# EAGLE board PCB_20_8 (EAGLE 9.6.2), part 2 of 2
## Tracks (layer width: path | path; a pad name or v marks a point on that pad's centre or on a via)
1PPS
  Top 0.406: U$1.4_TIMEPULSE 26.67,99.18 27.94,100.33 R703.2
+3V3  (via drill 0.3, 0.61)
  Top 0.152: IC800.57 IC800.58
  Top 0.254: v105.41,29.84 105.41,27.94 R825.2 | v105.41,37.47 107.95,37.47 | 114.16,61.42 IC800.19 | IC800.11 115.25,57.42 115.25,57.25 C805.1 | 97.37,52.42 IC800.75 | R821.1 85.41,57.47 v85.41,50.48 R822.1 | 111.76,87 111.76,87.02 | 114.94,60.64 C800.1 | v118.07,48.9 R803.2 120.44,41.35 BOOT0.1 | 99.41,60.96 99.41,60.92 IC800.58
  Top 0.305: 114.16,61.42 114.94,60.64 | v111.68,68.9 110.41,68.9 IC800.28 110.41,61.42 | 111.41,45.94 111.41,42.23 107.95,42.23 107.95,37.47 SERIAL.2 | 97.37,52.42 v97.37,50.48 C801.1 C817.1 97.37,40.01 SWD.1 | IC800.11 110.09,57.42 | 99.38,53.66 99.38,52.42 IC800.75 | 99.38,53.66 99.38,60.96 99.41,60.96 | 99.41,60.96 | 99.41,60.96 IC800.50 99.41,68.9 v98.42,68.9 C803.1 | IC800.19 110.41,61.42 | 110.09,53.66 110.49,53.34 111.41,52.42 IC800.100 v111.41,48.9 111.41,47.31 | 110.09,57.42 110.09,53.66 | 110.09,57.42 110.09,61.42 110.41,61.42 | 111.41,47.31 111.41,45.94 | 111.41,45.94 C802.1 | C804.1 111.76,68.9 | C815.1 111.76,71.12 | C816.1 111.51,47.41 111.41,47.31 | 110.09,53.66 99.38,53.66
  Top 0.406: 111.76,82.91 111.76,77.79 | 111.76,77.79 111.76,71.12 111.76,68.9 v111.68,68.9 | 111.76,82.91 111.76,87.02 IC502.3 | C510.1 111.76,87 | BOOT1.3 111.76,82.91 | F800.2 111.76,77.79
  Bottom 0.254: v105.41,29.84 v105.41,37.47 | v85.41,50.48 v97.37,50.48 | v118.07,48.9 v111.41,48.9
  Bottom 0.305: v111.68,68.9 v98.42,68.9 | BOOT0.2 BOOT0.1
  Bottom 0.406: BOOT1.4 BOOT1.3
+3V3-C  (via drill 0.61)
  Top 0.406: D3-C.2 v156.21,118.43 D4-C.2 | D6-C.2 v162.56,118.43 D5-C.2 | D1-C.2 v149.86,118.43 D2-C.2 | IC4.3 v162.88,104.14 162.24,105.41 IC3.7 | IC3.3 v153.03,104.14 152.4,105.41 IC2.7 | IC2.3 v142.56,104.14 142.56,92.98 C15.1 C9.1 147.64,90.79 IC5.5 | v172.72,104.14 172.72,105.41 IC4.7
  Bottom 0.406: v162.56,118.43 v156.21,118.43 153.67,118.43 | v172.72,104.14 v162.88,104.14 153.67,104.14 | 153.67,104.14 v153.03,104.14 v142.56,104.14 | v149.86,118.43 153.67,118.43 | 153.67,118.43 153.67,104.14
+3V3-E  (via drill 0.3, 0.5)
  Top 0.254: IC600.20 IC600.19
  Top 0.305: R607.2 101.6,100.75 v101.6,102.87
  Top 0.406: 86.36,115.25 v86.36,112.08 86.36,110.49 | 86.36,110.49 91.44,110.49 | v73.03,110.49 86.36,110.49 | v99.06,110.49 IC600.19 | IC600.25 91.44,110.49 | 91.44,110.49 v99.06,110.49 | v106.68,112.08 106.68,121.92 106.68,124.46 C606.2 IC504.3 | IC600.28 86.36,115.25 | 86.36,115.25 C604.2 | IC600.15 104.14,110.49 v101.6,110.49 v99.06,110.49 | F600.1 v43.18,110.49
  Bottom 0.305: v101.6,102.87 v101.6,110.49
  Bottom 0.406: v43.18,110.49 v73.03,110.49 | v106.68,112.08 v86.36,112.08
+3V3-G
  Top 0.406: F700.1 C518.1 45.24,104.87 IC505.3
+5V  (via drill 0.3 pad 0.25, 0.35, 0.6)
  Top 0.254: v59.05,12.38 C419.2 53.34,13.26 53.02,14.29 IC403.7 | IC303.7 53.02,35.24 | 53.02,56.52 IC203.7 | IC103.7 53.02,78.11
  Top 0.305: 53.02,35.24 53.34,34.21 C319.2 v59.05,33.34 59.05,30.58 C227.2 IC304.5 | 53.02,56.52 53.34,55.48 C219.2 v59.05,54.61 59.05,51.85 C327.2 IC204.5 | 53.02,78.11 53.34,77.08 C119.2 v59.05,76.2 59.05,73.44 C427.2 IC104.5 | v59.05,12.38 59.05,9.63 C127.2 IC404.5
  Top 0.406: v75.25,80.01 v75.25,70.8 v75.25,58.42 v75.25,37.15 v75.25,16.19 v75.25,12.7 v75.25,6.99 | v90.17,7.94 C513.1 97.16,7.95 IC503.5 | L403.1 v11.43,12.7 | v90.17,12.7 87.32,12.69 v86.36,12.7
  Bottom 0.305: v75.25,16.19 62.87,16.19 62.87,12.38 v59.05,12.38 | v59.05,33.34 62.87,33.34 62.87,37.15 v75.25,37.15 | v59.05,54.61 62.87,54.61 62.87,58.42 v75.25,58.42 | v59.05,76.2 62.87,76.2 62.87,80.01 v75.25,80.01
  Bottom 0.406: v75.25,70.8 16.51,70.8 H-INPUT.4 | H-INPUT.4 | v75.25,6.99 74.61,6.35 11.43,6.35 v11.43,12.7 | v86.36,12.7 | v75.25,12.7 | v86.36,12.7 v75.25,12.7 | v90.17,12.7 v90.17,7.94
A1
  Top 0.406: R17.1 R10.1 IC4.4
A2
  Top 0.406: R15.1 R8.1 IC3.4
A3
  Top 0.305: 146.05,102.73 IC2.4
  Top 0.406: R12.1 R7.1 146.05,102.73
ADA4891
  Top 0.406: IC1.1 160.66,26.04 160.66,27.94 IC1.4 R2.1 R5.1
AGND  (via drill 0.3, 0.5, 0.6, 0.6 pad 0.25)
  Top 0.254: IC103.3 IC103.2 53.02,86.04 54.61,87.23 C118.2 | 24.45,81.92 29.84,81.92 C105.1 30.8,79.38 32.07,79.38 | IC203.3 IC203.2 53.02,64.45 54.61,65.64 C218.2 | IC202.4 47.82,59.05 45.72,59.05 C214.2 44.45,57.7 v44.45,55.24 | 24.45,38.73 24.45,39.05 29.84,39.05 C305.1 30.8,36.51 32.07,36.51 | 24.45,38.73 C304.1 24.13,36.73 C300.2 C301.2 18.73,33.72 v18.73,33.34 17.78,32.38 R305.1 | R302.2 24.45,38.73 | C401.2 | C401.2 C400.2 24.13,15.77 C404.1 24.45,18.1 | C106.1 C107.1 39.05,71.75 43.5,71.75 R115.1 45.51,72.81 v45.72,73.03 | C406.1 C407.1 39.05,7.94 43.81,7.94 R415.1 46.26,9.27 v46.35,9.21 | C306.1 C307.1 39.05,28.89 43.5,28.89 R315.1 45.67,30.19 v45.72,30.16 | IC403.3 IC403.2 53.02,22.23 54.61,23.42 C418.2 | IC303.3 IC303.2 53.02,43.18 54.61,44.37 C318.2 | 56.83,84.77 v55.88,86.04 55.88,88.03 C118.2 | 56.83,41.91 v55.88,43.18 55.88,45.17 C318.2 | 56.83,20.95 v55.88,22.23 55.88,24.21 C418.2 | v63.5,84.77 56.83,84.77 | v63.5,63.18 56.83,63.18 | 56.83,63.18 v55.88,64.45 55.88,66.36 54.61,66.36 C218.2 | v63.5,41.91 56.83,41.91 | v63.5,20.95 56.83,20.95 | R105.1 17.78,75.25 v18.73,76.2 18.73,76.58 C101.2 C100.2 24.13,79.59 C104.1 24.45,81.92 | R205.1 17.78,53.66 v18.73,54.61 18.73,54.99 C201.2 C200.2 24.13,58 C204.1 24.45,60.01 | R309.1 32.07,36.51 | 32.07,36.51 36.51,36.51 | R310.1 38.73,36.51 36.51,36.51 | 36.51,36.51 R308.1 38.42,33.76 R311.1 38.73,33.97 40.96,33.97 | 24.45,60.01 24.45,60.33 29.84,60.33 C205.1 30.8,57.78 32.07,57.78 | 24.45,18.1 24.45,18.41 R402.2 | 24.45,18.1 30.8,18.1 C405.1 31.75,15.56 36.51,15.56 | R209.1 32.07,57.78 | 36.51,57.78 R208.1 38.42,55.03 R211.1 38.73,55.24 41.06,55.24
  Top 0.254: 36.51,57.78 32.07,57.78 | R210.1 38.73,57.78 36.51,57.78 | 36.51,79.38 R108.1 38.42,76.62 R111.1 38.73,76.83 41.06,76.83 | 36.51,79.38 32.07,79.38 | R109.1 32.07,79.38 | 36.51,79.38 38.73,79.38 R110.1 | 36.51,15.56 R408.2 38.42,13.02 41.06,13.02 | 36.51,15.56 38.73,15.56 R410.1 | R414.1 41.06,13.02 | 41.06,13.02 v44.45,13.02 | v44.45,55.24 41.06,55.24 | 41.06,55.24 R214.1 | C323.2 v63.5,41.91 | v63.5,41.91 C321.2 63.5,40.64 60.83,40.64 IC305.4 | v63.5,20.95 C421.2 63.5,19.61 60.83,19.61 IC405.4 | v63.5,20.95 C423.2 | R218.1 56.83,63.18 | R318.1 56.83,41.91 | R418.1 56.83,20.95 | v63.5,63.18 C221.2 63.5,61.91 60.83,61.91 IC205.4 | C223.2 v63.5,63.18 | R217.1 44.55,55.24 v44.45,55.24 | R202.2 24.45,60.01 | v45.72,51.44 45.67,51.47 R215.1 43.5,50.16 39.05,50.16 C207.1 C206.1 | C218.2 52.7,68.16 R216.1 | R316.1 52.7,46.89 C318.2 | IC302.4 47.82,37.78 46.04,37.78 46.04,36.51 45.72,36.51 | C314.2 45.72,36.51 | 45.72,36.51 44.45,36.51 v44.45,33.97 | v44.45,33.97 40.96,33.97 | R314.1 40.96,35.56 40.96,33.97 | v44.45,33.97 44.55,33.97 R317.1 | C118.2 52.7,89.75 R116.1 | 56.83,84.77 R118.1 | R416.1 52.7,25.93 C418.2 | IC105.4 60.83,83.5 63.5,83.5 | 63.5,83.5 C121.2 | 63.5,83.5 v63.5,84.77 | v63.5,84.77 C123.2 | v44.45,13.02 44.5,13.07 R417.1 | IC402.4 47.82,16.83 46.04,16.83 46.04,15.56 45.72,15.56 | 45.72,15.56 44.45,15.56 v44.45,13.02 | v44.45,76.83 41.06,76.83 | R114.1 41.06,76.83 | 24.45,81.92 24.45,82.23 R102.2 | C414.2 45.72,15.56 | R117.1 44.45,75.25 v44.45,76.83 | v44.45,76.83 44.45,79.29 C114.2 45.72,80.64 47.82,80.64 IC102.4 | C401.2 17.78,11.18 R405.2
  Top 0.406: v76.2,84.77 v76.2,63.18 v76.2,41.91 v76.2,20.95 | IC500.4 84.14,79.38 84.14,83.08 R502.1 v80.01,84.77
  Bottom 0.254: v45.72,51.44 45.72,53.98 v44.45,55.24 47.31,57.78 55.88,57.78 v55.88,64.45 | v55.88,86.04 55.88,79.38 47.31,79.38 v44.45,76.83 45.72,75.56 v45.72,73.03 | v46.35,9.21 46.35,11.11 v44.45,13.02 47.31,15.88 55.88,15.88 v55.88,22.23 | v45.72,30.16 45.72,32.7 v44.45,33.97 47.31,36.51 55.88,36.51 v55.88,43.18 | 18.73,48.26 v18.73,33.34 | 18.73,88.9 v18.73,76.2 | 18.73,59.69 v18.73,54.61
  Bottom 0.406: v63.5,84.77 v76.2,84.77 v80.01,84.77 | TR3.6 18.73,48.26 | TR2.6 18.73,59.69 | v63.5,63.18 v76.2,63.18 | v63.5,41.91 v76.2,41.91 | v63.5,20.95 v76.2,20.95 | TR1.6 18.73,88.9
AMP-CH1  (via drill 0.3)
  Top 0.254: IC800.16 v111.44,59.92 | v87.63,59.92 v87.63,84.45 | v83.4,84.45 C128.1
  Top 0.406: C128.1 L104.1
  Bottom 0.254: v87.63,84.45 v83.4,84.45 | v111.44,59.92 v87.63,59.92
AMP-CH2  (via drill 0.3)
  Top 0.254: IC800.34 107.41,67.94 v107.95,67.94 | v86.36,67.94 83.95,67.94 L204.1
  Top 0.406: C228.1 L204.1
  Bottom 0.254: v107.95,67.94 v86.36,67.94
AMP-CH3  (via drill 0.3)
  Top 0.254: L304.1 84.58,46.04 86.36,46.04 v86.36,63.5 | v107.91,63.5 IC800.33
  Top 0.406: C328.1 L304.1
  Bottom 0.254: v86.36,63.5 v107.91,63.5
AMP-CH4  (via drill 0.3)
  Top 0.254: v87.63,58.42 87.63,26.35 L404.1 | IC800.36 v106.41,58.42
  Top 0.406: L404.1 C428.1
  Bottom 0.254: v106.41,58.42 v87.63,58.42
BEEP  (via drill 0.3)
  Top 0.254: v125.73,95.25 R801.2 | IC800.30 109.41,70.17 v108.58,71.12
  Bottom 0.254: v125.73,95.25 125.73,71.12 v108.58,71.12
BNC2A  (via drill 0.3)
  Top 0.254: 64.77,88.3 IC106.3 v65.72,90.17 | 64.77,88.3 63.5,88.3 C123.1 | R119.2 62.87,79.38 64.77,80.64 64.77,88.3 | L104.2 v79.06,90.17
  Bottom 0.254: v65.72,90.17 v79.06,90.17
BNC2B  (via drill 0.3)
  Top 0.254: 64.77,66.71 64.77,59.05 62.87,57.78 R219.2 | C223.1 63.5,66.71 64.77,66.71 | v79.06,68.58 L204.2 | 64.77,66.71 IC206.3 v65.72,68.58
  Bottom 0.254: v65.72,68.58 v79.06,68.58
BNC2D  (via drill 0.3)
  Top 0.254: R419.2 62.87,15.56 64.77,16.83 64.77,24.48 | 64.77,24.48 IC406.3 v65.72,26.35 | 64.77,24.48 63.5,24.48 C423.1 | v79.06,26.35 L404.2
  Bottom 0.254: v79.06,26.35 v65.72,26.35
BOOT1
  Top 0.254: IC800.37 105.91,76.2
  Top 0.406: R818.2 105.91,76.2 105.91,78.38 BOOT1.1
  Bottom 0.406: BOOT1.2 BOOT1.1
C106
  Top 0.254: R107.1 C103.2 21.91,74.51 R106.1 R105.2 15.88,72.81 | R101.1 15.88,78.21
  Top 0.406: 15.88,72.81 15.88,78.21 15.88,83.19 TR1.4
CLK1
  Top 0.254: IC103.5 49.85,79 49.85,73.34 IC104.4
CLK1I  (via drill 0.3)
  Top 0.254: IC104.2 v51.44,71.75 | IC800.40 104.41,70.17 v102.87,71.75
  Bottom 0.254: v51.44,71.75 v102.87,71.75
CLK2
  Top 0.254: IC204.4 49.85,51.75 49.85,57.47 50.48,57.47 IC203.5
CLK2I  (via drill 0.3)
  Top 0.254: IC204.2 v51.44,49.85 | IC800.96 109.41,49.56 v109.44,48.9
  Bottom 0.254: v51.44,49.85 109.22,49.85 v109.44,48.9
CLK3
  Top 0.254: IC303.5 49.85,36.13 49.85,30.48 IC304.4
CLK3I  (via drill 0.3)
  Top 0.254: IC304.2 v51.44,28.89 | v86.36,43.18 v86.36,28.89 | IC800.5 116.84,54.42 v116.84,43.18
  Bottom 0.254: v86.36,28.89 v51.44,28.89 | v116.84,43.18 v86.36,43.18
CLK4
  Top 0.254: IC403.5 49.85,15.18 49.85,9.53 IC404.4
CLK4I  (via drill 0.3)
  Top 0.254: IC404.2 v51.44,7.94 | v88.9,21.27 v88.9,56.92 | IC800.66 v94.61,56.92
  Bottom 0.254: v51.44,7.94 88.9,7.94 v88.9,21.27 | v88.9,56.92 v94.61,56.92
CS  (via drill 0.3)
  Top 0.254: v73.66,87.63 v73.66,66.04 v73.66,49.21 v73.66,44.77 v73.66,23.81 | IC205.6 61.32,65.72 v61.59,66.04 | v48.58,87.63 48.3,87.35 IC102.6 | v48.58,66.04 48.3,65.76 IC202.6 | v61.59,87.63 61.32,87.35 IC105.6 | IC302.6 48.3,44.49 v48.58,44.77 | IC305.6 61.32,44.49 v61.59,44.77 | IC402.6 48.3,23.53 v48.58,23.81 | IC405.6 61.32,23.53 v61.59,23.81 | IC800.2 114.94,52.92 v114.94,48.26
  Bottom 0.254: v48.58,87.63 v61.59,87.63 v73.66,87.63 | v48.58,66.04 v61.59,66.04 v73.66,66.04 | v48.58,44.77 v61.59,44.77 v73.66,44.77 | v73.66,23.81 v61.59,23.81 v48.58,23.81 | v73.66,49.21 80.01,49.21 80.01,48.26 v114.94,48.26
E-ANTENNE  (via drill 0.6)
  Top 0.406: IN.1 R1.2
  other vias: 156.21,71.12 156.21,64.77 156.21,58.42 156.21,52.07 163.83,52.07 163.83,58.42 171.45,71.12 171.45,64.77 171.45,58.42 171.45,52.07
  pour Bottom: 173.99,72.71 153.99,72.71 153.99,64.77 151.45,64.77 151.45,72.71 140.97,72.71 140.97,0 151.45,0 151.45,62.23 153.99,62.23 153.99,45.72 162.56,45.72 162.56,36.83 165.1,36.83 165.1,45.72 173.99,45.72
  pour Top: 153.99,45.72 162.56,45.72 162.56,36.83 165.1,36.83 165.1,45.72 173.99,45.72 173.99,72.71 153.99,72.71 153.99,64.77 151.45,64.77 151.45,72.71 140.97,72.71 140.97,0 151.45,0 151.45,62.23 153.99,62.23
ENC28J60-CS  (via drill 0.3)
  Top 0.254: v96.52,85.09 R830.2
  Top 0.406: IC600.9 v97.79,97.79
  Bottom 0.406: v97.79,97.79 97.79,85.09 v96.52,85.09
ENC28J60-INT  (via drill 0.3)
  Top 0.254: v91.44,88.9 v91.44,55.88 | v111.44,55.92 IC800.8
  Top 0.305: R610.2 v91.44,97.79
  Bottom 0.254: v91.44,55.88 109.22,55.88 v111.44,55.92
  Bottom 0.406: v91.44,97.79 v91.44,88.9
ENC28J60-INT-A
  Top 0.305: IC600.4 R610.1
ENC28J60-SCK  (via drill 0.3)
  Top 0.254: v95.25,86.36 R829.2
  Top 0.406: IC600.8 v96.52,97.79
  Bottom 0.406: v96.52,97.79 96.52,86.36 v95.25,86.36
ENC28J60-SI  (via drill 0.3)
  Top 0.254: v95.25,88.9 92.71,88.9 R828.2
  Top 0.406: IC600.7 v95.25,97.79
  Bottom 0.406: v95.25,97.79 v95.25,88.9
ENC28J60-SO  (via drill 0.3)
  Top 0.254: v93.98,87.63 93.98,63.42 IC800.53
  Top 0.305: v93.98,97.79 R611.2
  Bottom 0.406: v93.98,97.79 v93.98,87.63
ENC28J60-SO-A
  Top 0.305: IC600.6 R611.1
GND  (via drill 0.3, 0.3 pad 0.25, 0.35, 0.5, 0.5 pad 0.25, 1.27 pad 2.54, 1.6 pad 2.18)
  Top 0.61: v85.09,8.89 v82.55,8.89 81.28,8.89 v81.28,11.11 | 80.33,9.84 82.23,9.84 | v102.87,8.89 99.06,8.89 v99.06,11.43 | 98.11,9.84 100.01,9.84
  other vias: 24.77,121.28 20.64,60.33 20.64,39.05 20.64,18.1 58.42,38.42 47.62,30.16 44.45,43.5 39.69,13.97 47.62,9.21 50.8,38.73 50.8,17.78 50.8,81.6 44.45,64.77 66.04,81.28 58.42,81.28 66.04,17.46 40.01,34.92 44.77,59.05 40.01,77.79 30.48,54.93 47.62,51.44 47.62,73.03 6.35,57.15 50.8,60.01 58.42,59.69 34.92,65.41 34.92,61.59 39.37,61.91 41.91,62.55 66.04,59.69 40.01,56.2 58.42,65.41 104.14,99.06 58.42,44.13 58.42,87 66.04,38.42 44.45,86.36 30.48,76.52 20.64,81.92 44.45,22.54 58.42,17.46 44.77,80.64 58.42,23.18 30.48,33.66 30.48,12.7 44.77,37.78 44.77,16.83 34.92,87 34.92,83.19 34.92,44.13 34.92,40.32 34.92,23.18 34.92,19.37 39.69,12.06 40.01,33.02 40.01,54.29 40.01,75.88 41.91,84.14 41.91,41.27 41.27,19.68 36.83,107.95 78.74,22.54 126.36,58.42 98.42,66.67 115.25,65.09 92.71,107.63 111.44,58.74 78.74,39.37 105.41,54.61 108.58,61.59 123.19,68.58 108.58,57.15 93.34,124.46 104.78,38.73 78.74,64.77 100.33,107.63 118.11,19.05 127,73.66 62.23,80.64 62.23,59.05 62.23,37.78 62.23,16.83 94.61,61.28 90.17,32.38 114.3,66.99 114.3,72.71 111.44,54.29 130.81,120.65 100.33,32.38 120.65,80.64 134.62,86.36 134.62,80.01 113.67,51.44 118.11,51.44 90.17,22.86 95.25,116.84 101.6,54.61 101.6,61.59 129.54,19.05 6.35,45.72 6.35,86.36 82.55,100.33 78.74,31.75 129.54,30.48 88.9,107.63 102.87,124.46 124.46,120.65 101.6,88.9 105.41,88.9 101.6,92.71 101.6,96.52 90.17,38.73 100.33,38.73 124.46,110.49 90.17,26.04 121.92,26.67 110.49,48.9 96.2,52.39 101.6,52.7 105.41,52.7 108.58,52.7 126.36,51.44 101.6,57.15 105.41,57.15 108.58,54.61 111.44,63.5 101.6,64.45 104.78,61.59 104.78,64.45 104.78,71.75 100.33,116.84 129.54,26.67 125.73,19.05 78.74,19.05 86.36,22.86 90.17,19.05 114.94,41.91 21.59,96.52 120.65,102.87 86.36,19.05 100.33,8.89 114.3,80.64 120.65,83.82 114.3,83.82 117.47,83.82 90.17,15.24 78.74,15.24 82.55,19.05 83.82,11.11 86.36,15.24 105.41,92.71 109.22,92.71 82.55,15.24 97.16,12.7 107.31,12.06 101.92,11.43 2.54,51.44 47.62,101.6 111.76,117.79 71.12,107.95 119.7,93.98 123.83,93.98 102.23,80.64 97.79,76.2 100.33,76.2 78.74,35.56 118.11,54.61 120.02,60.96 113.03,88.9 109.22,96.52 86.36,64.77 82.55,39.37 82.55,35.56 82.55,31.75 78.74,42.55 125.73,30.48 116.2,33.02 121.92,77.47 19.68,109.86 114.94,117.79 108.58,117.79 114.94,114.62 108.58,114.62 50.8,101.6 44.45,101.6 44.45,96.2 50.8,96.2 67.31,107.95 96.52,116.84 134.62,110.49 71.12,104.14 74.93,104.14 78.74,104.14 82.55,104.14 82.55,92.71 79.38,92.71 78.74,100.33 67.31,121.92 67.31,125.73 67.31,116.84 71.12,116.84 74.93,121.92 59.69,121.92 59.69,125.73 59.69,116.84 52.07,125.73 55.88,125.73 44.45,107.95 74.93,100.33 74.93,107.95 63.5,107.95 44.45,121.92 44.45,125.73 44.45,116.84 52.07,121.92 55.88,116.84 40.64,107.95 78.74,106.68 82.55,106.68 71.12,100.33 67.31,100.33 63.5,100.33 33.02,121.92 33.02,125.73 48.26,121.92 48.26,125.73 48.26,116.84 52.07,116.84 55.88,121.92 48.26,107.95 63.5,121.92 63.5,125.73 63.5,116.84 71.12,121.92 74.93,116.84 78.74,121.92 78.74,125.73 78.74,116.84 71.12,125.73 74.93,125.73 86.04,121.92 86.04,125.73 86.04,116.84 82.23,125.73 55.88,107.95 59.69,107.95 52.07,107.95 82.23,121.92 82.23,116.84 40.64,116.84 40.64,121.92 29.21,116.84 36.83,121.92 36.83,116.84 86.36,92.71 102.87,121.92 74.93,92.71 52.07,92.71 71.12,92.71 102.87,119.38 55.88,92.71 63.5,92.71 67.31,92.71 59.69,92.71 48.26,92.71 105.41,96.52 113.03,92.71 109.22,88.9 17.78,107.95 25.4,107.95 21.59,107.95 29.21,107.95 33.02,107.95 13.97,107.95 6.35,107.95 2.54,107.95 17.78,104.14 17.78,96.52 21.59,104.14 10.16,92.71 13.97,92.71 17.78,92.71 21.59,100.33 2.54,104.46 82.55,96.52 86.36,96.52 86.36,88.9 79.38,96.52 55.88,96.52 74.93,96.52 59.69,96.52 67.31,96.52 71.12,96.52 63.5,96.52 71.12,111.76 67.31,111.76 44.45,111.76 74.93,111.76 63.5,111.76 48.26,111.76 55.88,111.76 59.69,111.76 52.07,111.76 33.02,111.76 83.82,6.67 81.28,6.67 113.03,96.52 116.84,96.52 116.84,100.33 113.03,100.33 109.22,100.33 116.84,92.71 116.84,88.9 120.65,96.52 120.65,100.33 124.46,96.52 101.6,85.09 105.41,85.09 109.22,85.09 109.22,78.42 8.6,79.5 8.6,64.01 105.41,19.05 112.08,19.05 133.35,11.43 121.92,19.05 133.35,7.62 129.54,11.43 125.73,26.67 118.11,26.67 125.73,15.24 125.73,22.86 108.58,19.05 121.92,15.24 129.54,7.62 121.92,30.48 13.97,7.62 13.97,26.67 13.97,15.24 118.11,15.24 118.11,7.62 114.3,7.62 121.92,7.62 125.73,7.62 129.54,15.24
  pour Bottom: 138.43,127 138.43,3.17 0,3.17 0,127
  pour Top: 138.43,127 0,127 0,3.17 138.43,3.17
GND-B  (via drill 0.3)
  other vias: 160.66,29.21 163.51,29.21 164.78,26.04 160.66,34.92 167.96,18.73 158.12,29.21 167.96,29.21 168.28,26.04
  pour Bottom: 173.99,43.18 173.99,0 153.99,0 153.99,43.18 161.93,43.18 161.93,36.2 165.74,36.2 165.74,43.18
  pour Top: 173.99,0 173.99,43.18 165.74,43.18 165.74,36.2 161.93,36.2 161.93,43.18 153.99,43.18 153.99,0
GND-C  (via drill 0.3, 1.6 pad 2.18)
  other vias: 155.26,113.03 163.83,113.03 145.41,113.03 162.88,101.92 153.03,101.92 143.83,101.92 172.72,107.95 162.24,107.95 152.4,107.95 148.27,113.03 158.12,113.03 167.64,113.03 165.1,119.38 158.75,119.38 152.4,119.38 160.66,95.25 168.28,95.25 154.31,95.25 157.48,95.25 151.76,95.25 165.74,95.25 149.86,90.17 165.1,90.17 149.7,86.23 165.23,86.26
  pour Bottom: 173.99,130.18 173.99,75.25 140.97,75.25 140.97,130.18
  pour Top: 173.99,75.25 173.99,130.18 140.97,130.18 140.97,75.25
GPS-1PPS  (via drill 0.3)
  Top 0.254: IC800.24 117.16,63.92 v117.16,69.85 | IC800.48 100.41,69.53 v100.73,69.85
  Top 0.406: R703.1 34.29,100.33 v35.56,99.06 | v88.9,97.79 v88.9,69.85
  Bottom 0.406: v35.56,99.06 88.9,99.06 v88.9,97.79 | v88.9,69.85 v100.73,69.85 v117.16,69.85
GPS-RX  (via drill 0.3)
  Top 0.254: IC800.25 116.2,64.42 v116.2,73.66 | IC800.35 v106.91,73.66
  Top 0.406: R701.1 v35.56,97.79 | v78.11,97.79 v78.11,73.66
  Bottom 0.254: v116.2,73.66 v106.91,73.66 v78.11,73.66
  Bottom 0.406: v78.11,97.79 v35.56,97.79
GPS-TX  (via drill 0.3)
  Top 0.254: v104.91,48.9 IC800.87
  Top 0.406: R700.1 v35.56,95.25 | v90.17,95.25 v90.17,48.9
  Bottom 0.406: v35.56,95.25 v90.17,95.25 | v90.17,48.9 v104.91,48.9
GPS-VCC
  Top 0.406: U$1.9_RESET_N 24.64,104.78 26.35,104.78 26.35,103.61 | 26.35,103.61 26.35,103.5 | 26.35,103.5 26.35,102.55 | 26.35,102.55 26.35,101.38 U$1.6_V_BCKP | U$1.7_VCC_IO 24.64,102.55 26.35,102.55 | U$1.8_VCC 24.64,103.5 26.35,103.5 | 26.35,103.61 C701.2 C700.2 R705.2
I1A  (via drill 0.61)
  Top 0.406: R18.2 v151.45,113.67 153.67,113.67 153.67,120.97 | 153.67,120.97 153.67,123.51 148.59,123.51 147.01,125.09 X1.2 | D2-C.3 153.67,120.97
  Bottom 0.406: SJ1.2 149.22,113.67 v151.45,113.67
I1B
  Top 0.406: R19.2 R25.1 147,113.35 147.96,114.3 147.96,116.52 | D1-C.3 147.96,116.52 | X1.1 143.51,124.14 147.96,119.7 147.96,116.52
I2A  (via drill 0.61)
  Top 0.406: R21.2 161.29,113.67 v160.02,113.67 160.02,120.97 | D4-C.3 160.02,120.97 | X1.5 157.51,124.75 160.02,122.24 160.02,120.97
  Bottom 0.406: SJ2.2 159.07,113.67 v160.02,113.67
I2B
  Top 0.406: R20.2 R26.1 156.84,113.67 154.94,115.57 154.94,116.52 | 154.94,116.52 154.94,126.27 X1.4 | D3-C.3 154.94,116.52
I3A  (via drill 0.61)
  Top 0.406: 166.37,120.97 166.37,123.51 168.01,125.14 X1.8 | 166.37,120.97 166.37,116.52 168.91,113.35 v171.13,113.35 R23.2 | D6-C.3 166.37,120.97
  Bottom 0.406: SJ3.2 168.91,113.35 v171.13,113.35
I3B
  Top 0.406: R22.2 R27.1 166.69,112.08 165.1,113.98 162.88,113.98 161.29,115.57 161.29,116.52 | 161.29,116.52 161.29,123.51 163.19,123.51 164.51,124.82 X1.7 | D5-C.3 161.29,116.52
IC202  (via drill 0.3)
  Top 0.254: IC205.3 v60.33,55.88 | R217.2 47.94,53.34 C216.2 v49.21,55.88
  Bottom 0.254: v60.33,55.88 v49.21,55.88
IC504IN
  Top 0.406: C515.1 114.07,124.46 IC504.1 116.84,120.99 116.84,110.49 114.56,110.49 | C514.1 114.56,110.49 | 114.56,110.49 R506.2
N$1
  Top 0.406: R501.1 C505.1 | C505.1 R500.2 | IC500.3 C505.1
N$2
  Top 0.254: IC100.1 19.37,85.41 19.37,84.45 19.65,84.45 R103.1 R104.1
N$3
  Top 0.254: IC205.2 59.82,61.91 58.1,61.91 R218.2 C220.2
N$4  (via drill 0.3)
  Top 0.254: IC105.3 v60.33,77.47 | R117.2 C116.2 v49.21,77.47
  Bottom 0.254: v60.33,77.47 v49.21,77.47
N$5
  Top 0.254: IC106.4 65.72,87 68.58,87 R121.1
N$6
  Top 0.254: R103.2 24.34,84.14 R102.1 21.29,82.89 IC100.4
N$7
  Top 0.254: R111.2 40.01,79.27 40.01,82.87 | R112.1 40.01,82.87 | IC101.4 40.01,85.09 40.01,82.87
N$8
  Top 0.254: IC105.2 59.82,83.5 58.1,83.5 R118.2 C120.2
N$9
  Top 0.406: R503.1 LED1.A
N$10
  Top 0.254: IC800.13 120.02,58.42 Q2.2
  Top 0.406: Q2.2 123.51,62.76 C813.2
N$11
  Top 0.254: L401.2 L402.1 C406.2
N$12
  Top 0.406: IC500.1 R502.2
N$13
  Top 0.254: R119.1 59.33,79.42 IC105.1
N$14
  Top 0.254: IC402.2 46.8,19.68 43.81,19.68 43.81,17.78 C413.2 R414.2
N$15
  Top 0.254: IC305.2 59.82,40.64 58.1,40.64 R318.2 C320.2
N$16
  Top 0.254: R219.1 59.33,57.83 IC205.1
N$17
  Top 0.254: R207.1 C203.2 21.91,52.92 R206.1 R205.2 15.24,51.22 | R201.1 15.24,56.62
  Top 0.406: 15.24,51.22 TR2.4 15.24,56.62
N$18
  Top 0.254: C208.1 C207.2 38.83,52.72 R208.2 36.2,55.03 C209.1 33.34,55.05 L202.2
N$19
  Top 0.254: C205.2 28.02,56.15 L200.2 L201.1
N$20
  Top 0.254: IC305.1 59.33,36.51 R319.1
N$21
  Top 0.254: L301.2 L302.1 C306.2
N$22
  Top 0.254: IC202.2 46.8,61.91 46.35,61.91 43.81,61.91 43.81,60.01 C213.2 R214.2
N$23
  Top 0.254: R209.2 C209.2 36.2,58.84 C210.1
N$24
  Top 0.254: 34.29,64.35 34.29,60.54 C210.2 | 34.29,64.35 34.29,68.16 R213.1 | C211.1 34.29,64.35
N$25
  Top 0.406: SMA20.SIG 26.89,65.09 C229.1
N$26
  Top 0.254: R313.2 38.7,44.13 IC301.1 40.32,44.13 40.32,43.18 42.76,43.18 R312.2 41.06,38.1 C313.1
N$27
  Top 0.254: R419.1 59.33,15.56 IC405.1
N$28
  Top 0.254: R210.2 38.73,62.65 | 38.73,62.65 38.73,63.5 IC201.3 | C211.2 38.73,62.65
N$29
  Top 0.254: IC200.1 19.37,63.82 19.37,62.87 R203.1 R204.1
N$30  (via drill 0.3)
  Top 0.254: C308.2 41.8,29.95 R315.2 v43.5,33.02 | v44.77,41.59 47.31,41.59 IC302.3
  Bottom 0.254: v43.5,33.02 43.5,41.59 v44.77,41.59
N$31
  Top 0.254: L200.1 C204.2 24.45,53.98 20,53.98 R206.2
N$32
  Top 0.254: C124.2 R120.2
N$33
  Top 0.254: IC201.4 40.01,63.5 40.01,61.28 | 40.01,61.28 R212.1 | R211.2 40.01,58 40.01,61.28
N$34
  Top 0.254: R203.2 24.34,62.55 R202.1 21.29,61.3 IC200.4
N$35
  Top 0.406: R606.2 IC600.14
N$36
  Top 0.254: R120.1 R121.2 71.65,89.53 68.26,89.53 IC106.1
N$37
  Top 0.254: C213.1 41.06,59.37 R212.2 42.76,64.45 40.64,64.45 40.64,65.4 IC201.1 R213.2
N$38  (via drill 0.3)
  Top 0.254: C208.2 41.8,51.22 R215.2 v43.5,54.29 | IC202.3 47.31,62.87 v44.77,62.87
  Bottom 0.254: v43.5,54.29 43.5,62.87 v44.77,62.87
N$39
  Top 0.254: C113.1 41.06,80.96 R112.2 42.76,86.04 40.32,86.04 40.32,86.99 IC101.1 R113.2
N$40
  Top 0.254: IC405.2 59.82,19.68 58.1,19.68 R418.2 C420.2
N$41
  Top 0.406: SMA11.SIG 71.75,75.88 C124.1
N$42
  Top 0.254: L302.2 33.34,33.78 C309.1 36.2,33.76 R308.2 38.83,31.44 C307.2 C308.1
N$43
  Top 0.254: L301.1 L300.2 28.02,34.88 C305.2
N$44
  Top 0.254: L400.1 26.38,16 C404.2 24.45,11.75 20,11.75 R406.2
N$45
  Top 0.406: IC600.24 92.71,118.43 Q1.1 89,121.92 C603.2
N$46
  Top 0.254: R314.2 C313.2 43.81,38.73 43.81,40.64 46.8,40.64 IC302.2
N$47
  Top 0.254: R309.2 C309.2 36.2,37.57 C310.1
N$48
  Top 0.254: R313.1 34.29,46.89 34.29,43.08 | 34.29,43.08 34.29,39.27 C310.2 | C311.1 34.29,43.08
N$49
  Top 0.254: R413.2 38.7,23.18 IC401.1 40.32,23.18 40.32,22.23 42.86,22.23 42.86,21.27 | IC401.4 42.86,21.27 | 42.86,21.27 42.86,18.73 C413.1
N$50
  Top 0.254: 38.73,41.38 38.73,42.23 IC301.3 | 38.73,41.38 R310.2 | C311.2 38.73,41.38
N$51
  Top 0.406: SMA40.SIG 26.99,22.86 C429.1
N$52
  Top 0.254: C329.2 23.32,45.27 R304.2
N$53
  Top 0.254: 40.01,40.01 40.01,36.73 R311.2 | 40.01,40.01 40.01,42.23 IC301.4 | R312.1 40.01,40.01
N$54
  Top 0.254: R407.1 C403.2 21.91,10.69 R406.1 R405.1 16.19,8.99 16.19,11.43 16.19,14.39 R401.1
  Top 0.305: C430.2 16.19,11.43
N$55  (via drill 0.3 pad 0.25)
  Top 0.254: v50.48,64.45 50.16,64.77 C217.1 | v49.21,59.05 C216.1 | v44.77,60.33 46.32,60.33 IC202.1
  Bottom 0.254: v44.77,60.33 49.21,60.33 | v49.21,59.05 49.21,60.33 | 49.21,60.33 v50.48,64.45
N$56
  Top 0.254: L201.2 L202.1 C206.2
N$57
  Top 0.254: R304.1 R303.1 19.37,41.59 19.37,42.54 IC300.1
N$58
  Top 0.254: C224.2 R220.2
N$59
  Top 0.254: L401.1 L400.2 C405.2
N$60
  Top 0.406: SMA21.SIG 71.75,54.29 C224.1
N$61
  Top 0.406: IC600.23 93.98,118.43 Q1.2 97.69,121.92 C602.2
N$62
  Top 0.254: R220.1 R221.2 71.65,67.94 68.26,67.94 IC206.1
N$63
  Top 0.254: C324.2 R320.2
N$64  (via drill 0.3)
  Top 0.254: C408.1 C407.2 38.83,10.49 R408.1 v34.61,14.29 L402.2 | C410.1 36.51,16.83 v34.61,16.83
  Bottom 0.254: v34.61,16.83 v34.61,14.29
N$65
  Top 0.254: R413.1 34.29,25.93 34.29,22.12 | 34.29,22.12 34.29,18.31 C410.2 | C411.1 34.29,22.12
N$66
  Top 0.254: R420.1 R421.2 71.65,25.72 68.26,25.72 IC406.1
N$67
  Top 0.254: R410.2 38.73,20.42 | 38.73,20.42 38.73,21.27 IC401.3 | C411.2 38.73,20.42
N$68
  Top 0.254: L101.2 L102.1 C106.2
N$69  (via drill 0.3)
  Top 0.254: R600.1 v30.48,119.06 | IC600.27 v88.9,119.06
  Bottom 0.254: v88.9,119.06 v30.48,119.06
N$70  (via drill 0.3)
  Top 0.254: C408.2 42.12,8.99 R415.2 v43.81,12.06 | IC402.3 47.31,20.64 v44.77,20.64
  Bottom 0.254: v43.81,12.06 43.81,20.64 v44.77,20.64
N$71
  Top 0.254: R320.1 R321.2 71.65,46.67 68.26,46.67 IC306.1
N$72
  Top 0.406: R100.2 3.17,88.9 TR1.1
  Bottom 0.406: TR1.1 12.38,88.9 12.38,76.2 H-INPUT.1
N$73
  Top 0.406: R100.1 3.17,83.82 TR1.3
  Bottom 0.406: TR1.3 10.48,83.82 10.48,74.93 H-INPUT.2
N$74
  Top 0.406: R200.2 3.17,59.69 TR2.1
  Bottom 0.406: H-INPUT.3 9.53,73.66 9.53,66.36 10.48,66.36 10.48,59.69 TR2.1
N$75
  Top 0.406: R200.1 3.17,54.61 TR2.3
  Bottom 0.406: H-INPUT.6 10.48,69.85 10.48,67.31 11.43,67.31 11.43,54.61 TR2.3
N$76
  Top 0.406: R300.2 3.17,48.26 TR3.1
  Bottom 0.406: H-INPUT.7 12.38,68.58 12.38,48.26 TR3.1
N$77
  Top 0.406: R300.1 3.17,43.18 TR3.3
  Bottom 0.406: H-INPUT.8 13.34,67.31 13.34,43.18 TR3.3
N$78
  Top 0.254: R303.2 24.34,41.27 R302.1 21.29,40.03 IC300.4
N$79
  Top 0.406: R600.2 30.48,126.36 3.3,126.36 RJ1.G+
N$80  (via drill 0.3)
  Top 0.254: C108.2 41.8,72.81 R115.2 v43.5,75.88 | IC102.3 47.31,84.45 v44.77,84.45
  Bottom 0.254: v43.5,75.88 43.5,84.45 v44.77,84.45
N$81
  Top 0.254: R404.1 R403.1 19.37,20.64 19.37,21.59 IC400.1
N$82  (via drill 0.3)
  Top 0.254: R601.1 v27.94,118.11 | IC600.26 v90.17,116.84
  Bottom 0.254: v27.94,118.11 90.17,118.11 v90.17,116.84
N$83  (via drill 0.3)
  Top 0.254: IC203.1 v54.29,64.45 | v52.07,64.45 R216.2 52.07,66.46 C217.2
  Bottom 0.254: v54.29,64.45 v52.07,64.45
N$84
  Top 0.254: C220.1 54.29,57.23 IC203.8
N$85
  Top 0.254: R113.1 34.29,89.75 34.29,85.94 | 34.29,85.94 34.29,82.13 C110.2 | C111.1 34.29,85.94
N$86
  Top 0.254: R403.2 24.34,20.32 R402.1 21.29,19.07 IC400.4
N$87  (via drill 0.3)
  Top 0.254: v52.07,86.04 R116.2 52.07,88.05 C117.2 | v54.29,86.04 IC103.1
  Bottom 0.254: v52.07,86.04 v54.29,86.04
N$88
  Top 0.254: R307.1 C303.2 21.91,31.65 R306.1 R305.2 15.24,29.95 | R301.1 15.24,35.34
  Top 0.406: TR3.4 15.24,35.34 15.24,29.95
N$89
  Top 0.254: IC101.3 38.73,85.09 38.73,84.24 | 38.73,84.24 R110.2 | C111.2 38.73,84.24
N$90
  Top 0.254: IC103.8 54.29,78.79 C120.1
N$91
  Top 0.254: L102.2 33.34,76.64 C109.1 36.2,76.62 R108.2 38.83,74.31 C107.2 C108.1
N$92
  Top 0.254: L101.1 L100.2 28.02,77.74 C105.2
N$93  (via drill 0.3)
  Top 0.254: C317.1 50.16,43.5 v50.48,43.18 | C316.1 v49.21,37.78 | v44.77,39.05 46.32,39.05 IC302.1
  Bottom 0.254: v50.48,43.18 49.21,39.05 | 49.21,39.05 v49.21,37.78 | v44.77,39.05 49.21,39.05
N$94
  Top 0.254: IC102.2 46.8,83.5 43.81,83.5 43.81,81.6 C113.2 R114.2
N$95  (via drill 0.3)
  Top 0.254: IC305.3 v60.33,34.61 | v49.21,34.61 47.94,34.61 C316.2 R317.2
  Bottom 0.254: v60.33,34.61 v49.21,34.61
N$96
  Top 0.254: C110.1 36.2,80.43 C109.2 R109.2
N$97
  Top 0.254: 4.83,109.92 arc90 5.08,110.17
  Top 0.406: R601.2 27.94,125.09 13.97,125.09 10.16,118.75 5.08,118.75 5.08,110.17 | RJ1.Y+ 4.83,109.92
N$98  (via drill 0.3)
  Top 0.254: C117.1 50.16,86.36 v50.48,86.04 | C116.1 v49.21,80.64 | v44.77,81.92 46.32,81.92 IC102.1
  Bottom 0.254: v49.21,80.64 49.21,81.92 | 49.21,81.92 v44.77,81.92 | 49.21,81.92 v50.48,86.04
N$99  (via drill 0.3)
  Top 0.254: C317.2 52.07,45.19 R316.2 v52.07,43.18 | v54.29,43.18 IC303.1
  Bottom 0.254: v52.07,43.18 v54.29,43.18
N$100
  Top 0.254: C320.1 54.29,35.95 IC303.8
N$101
  Top 0.305: IC600.1 C605.2
N$102  (via drill 0.3)
  Top 0.254: C416.1 v49.21,16.83 | C417.1 50.16,22.54 v50.48,22.23 | v44.77,18.1 46.32,18.1 IC402.1
  Bottom 0.254: v44.77,18.1 49.21,18.1 | 49.21,18.1 v49.21,16.83 | v50.48,22.23 49.21,18.1
N$103  (via drill 0.3)
  Top 0.254: IC405.3 v60.33,13.65 | v49.21,13.65 48.26,13.65 C416.2 R417.2
  Bottom 0.254: v60.33,13.65 v49.21,13.65
N$104  (via drill 0.3)
  Top 0.254: C417.2 52.07,24.23 R416.2 v52.07,22.23 | v54.29,22.23 IC403.1
  Bottom 0.254: v52.07,22.23 v54.29,22.23
N$105
  Top 0.254: C420.1 54.29,15 IC403.8
N$106
  Top 0.254: C104.2 | L100.1 C104.2 | R106.2 20,75.56 24.45,75.56 C104.2
N$107
  Top 0.254: C424.2 R420.2
N$108
  Top 0.406: IC600.10 R607.1
N$109
  Top 0.406: SMA41.SIG 71.75,12.06 C424.1
N$110  (via drill 0.3)
  Top 0.305: R603.2 R602.2 v20,115.25
  Top 0.406: R609.2 31.75,110.49 | 31.75,110.49 R608.2 | 31.75,110.49 29.31,110.49 C607.1 27.09,110.59 26.35,109.86 C600.2 R603.2
  Bottom 0.305: RJ1.P4 20,117.16 v20,115.25
N$111
  Top 0.254: L300.1 C304.2 | C304.2 | C304.2 24.45,32.7 20,32.7 R306.2
N$112  (via drill 0.3)
  Top 0.254: IC600.17 v101.6,113.03 | v29.21,114.3 v24.77,114.3 24.77,112.39 R603.1
  Bottom 0.254: v101.6,113.03 79.69,113.03 79.69,114.3 v29.21,114.3 | v24.77,114.3 24.77,118.43 16.19,118.43 RJ1.TD+
N$113  (via drill 0.3)
  Top 0.254: R602.1 v26.67,114.94 v26.67,119.7 | IC600.16 v102.87,113.67
  Bottom 0.254: v26.67,119.7 RJ1.TD- | v26.67,114.94 80.33,114.94 80.33,113.67 v102.87,113.67
N$114
  Top 0.406: SMA10.SIG 26.99,86.68 C129.1
N$115
  Top 0.406: C703.1 R704.2 19.68,93.34 19.68,100.34 U$1.14_VCC_RF R702.2 9.53,100.55 9.53,96.42 C702.1
N$116  (via drill 0.3)
  Top 0.254: IC600.12 101.6,108.58 v96.52,108.58 | v25.4,117.47 R604.2 23.07,116.2 19.37,116.2 RJ1.RD-
  Bottom 0.254: v96.52,108.58 78.42,108.58 78.42,113.03 25.4,113.03 v25.4,117.47
N$117  (via drill 0.3)
  Top 0.254: IC600.13 102.87,109.22 v97.79,109.22 | RJ1.RD+ 19.37,118.43 19.37,123.83 23.07,123.83 | 23.07,123.83 26.04,123.83 v26.04,115.89 | R605.2 23.07,123.83
  Bottom 0.254: v97.79,109.22 79.06,109.22 79.06,113.67 26.04,113.67 v26.04,115.89
N$118
  Top 0.254: R604.1 C601.2 R605.1
N$119
  Top 0.406: 120.65,107.95 128.27,107.95 R800.1 | BUZZER.+ 120.65,107.95 | T1.3 120.5,107.95 120.65,107.95
N$120
  Top 0.305: 125.73,104.14 R802.2
  Top 0.406: R802.2 R801.1 | T1.1 125.73,104.14
N$121
  Top 0.254: IC800.12 120.02,57.92 Q2.1
  Top 0.406: Q2.1 123.83,54.08 C814.2
N$122
  Top 0.406: 86.04,9.83 86.04,7.95 IC501.1 | IC501.3 86.04,9.83 | C502.1 88.9,9.83 | 88.9,9.83 86.04,9.83 | R508.2 R511.2 103.19,22.76 C503.1 103.08,19.05 94.61,19.05 94.61,9.83 88.9,9.83
N$123
  Top 0.406: R806.1 LED5.A
N$124
  Top 0.254: IC206.4 65.72,65.41 68.58,65.41 R221.1
N$125
  Top 0.406: IC505.1 53.98,104.8 | 53.98,104.8 57.78,104.8 | 57.78,104.8 60.7,104.8 R507.2 | C516.1 57.78,104.8 | C517.1 53.98,104.8
N$126  (via drill 0.3)
  Top 0.254: IC800.55 93.22,62.42 v92.71,60.96 | v78.74,60.96 J1.1
  Top 0.406: R821.2 J1.1
  Bottom 0.254: v92.71,60.96 v78.74,60.96
N$127  (via drill 0.3)
  Top 0.254: IC800.59 95.98,60.42 v93.34,57.78 | v78.74,57.78 78.74,53.98 J0.1
  Top 0.406: J0.1 R822.2
  Bottom 0.254: v93.34,57.78 v78.74,57.78
N$128
  Top 0.254: IC306.4 65.72,44.13 68.58,44.13 R321.1
N$129
  Top 0.406: R808.1 LED4.A
N$130
  Top 0.406: R812.1 LED3.A
N$131
  Top 0.406: C329.1 26.99,43.81 SMA30.SIG
N$132
  Top 0.254: C429.2 23.32,24.31 R404.2
N$133
  Top 0.254: C229.2 23.32,66.54 R204.2
N$135  (via drill 0.3)
  Top 0.254: IC800.26 113.03,66.02 v113.03,66.04 | v133.35,68.58 133.35,70.7
  Top 0.406: 133.35,70.7 R823.2 R824.1
  Bottom 0.254: v113.03,66.04 133.35,66.04 v133.35,68.58
N$136
  Top 0.254: IC406.4 65.72,23.18 68.68,23.18 R421.1
N$137
  Top 0.406: SMA31.SIG 71.75,33.02 C324.1
N$138
  Top 0.406: R816.1 LED2.A
N$139  (via drill 0.3, 0.5)
  Top 0.254: IC800.77 99.91,46.35 v100.55,45.72
  Top 0.406: R812.2 v134.62,46.67 R813.2
  Bottom 0.254: v100.55,45.72 134.62,45.72 v134.62,46.67
N$140  (via drill 0.3)
  Top 0.254: v131.44,45.09 131.44,35.14 R817.2 R816.2 | IC800.3 115.89,53.42 v115.89,45.09
  Bottom 0.254: v115.89,45.09 v131.44,45.09
N$141
  Top 0.406: R702.1 U$1.15_V_ANT/RESERVED
N$142
  Top 0.406: C7.1 156.53,19.05 L1.2 160.34,15.6 OUT.1
N$143
  Top 0.406: R5.2 C7.2
N$144
  Top 0.406: C2.1 IC1.3 R3.2
N$145
  Top 0.406: C1.1 C2.2 R2.2
N$146
  Top 0.254: C129.2 23.09,88.68 R104.2
N$147
  Top 0.813: U$1.11_RF_IN 6.74,103.58 arc90 4.45,101.28 GPS-IN.SIG
N$148
  Top 0.254: IC800.22 118.11,62.92 118.11,67.31 C807.2
  Top 0.406: C807.2 C809.2 R804.1 R831.1 R826.1
N$149  (via drill 0.3)
  Top 0.254: 131.44,55.46 v131.44,46.35 | IC800.81 101.91,47.94 v101.59,47.62
  Top 0.406: 131.44,55.46 R809.2 R808.2
  Bottom 0.254: v131.44,46.35 102.87,46.35 v101.59,47.62
N$150
  Top 0.254: IC800.49 99.91,70.48 100.97,71.28 C810.1
N$151
  Top 0.406: LED1B.A R504.1
N$152  (via drill 0.3)
  Top 0.254: IC800.83 102.91,47.59 105.13,45.36 v105.13,44.45 | 130.81,65.62 v130.81,44.45
  Top 0.406: 130.81,65.62 R807.2 R806.2
  Bottom 0.254: v105.13,44.45 v130.81,44.45
N$153
  Top 0.254: C811.1 95.25,53.02 95.65,53.42 IC800.73
N$154  (via drill 0.3)
  Top 0.254: IC800.94 108.41,48.9 108.58,48.58 R805.2 110.17,46.89 v110.17,43.81
  Bottom 0.254: v110.17,43.81 118.07,43.81 BOOT0.3
  Bottom 0.305: BOOT0.3 BOOT0.4
N$155
  Top 0.406: R814.1 LED7.A
N$156
  Top 0.406: R810.1 LED6.A
N$157  (via drill 0.3)
  Top 0.254: 129.54,74.3 v129.54,47.62 | v104.05,47.62 103.41,48.26 IC800.84
  Top 0.406: 129.54,74.3 130.81,74.3 130.81,102.77 132.08,102.77 132.08,106.26 R815.2 R814.2
  Bottom 0.254: v129.54,47.62 v104.05,47.62
N$158  (via drill 0.3)
  Top 0.254: 130.18,73.66 v130.18,46.99 | IC800.85 103.91,48.9 104.86,47.94 v104.86,46.99
  Top 0.406: 130.18,73.66 131.44,73.66 131.44,96.1 R811.2 R810.2
  Bottom 0.254: v130.18,46.99 v104.86,46.99
N$159
  Top 0.406: SERIAL.3 R819.2
N$160
  Top 0.406: R820.2 SERIAL.4
N$161  (via drill 0.3)
  Top 0.254: IC800.68 92.71,55.92 91.44,54.61 v91.44,40.64
  Bottom 0.254: J3.2 v91.44,40.64
N$162
  Top 0.406: R817.1 LED2B.A
N$163
  Top 0.406: R813.1 LED3B.A
N$164
  Top 0.406: R811.1 LED6B.A
N$165
  Top 0.406: R815.1 LED7B.A
N$166
  Top 0.406: R809.1 LED4B.A
N$167
  Top 0.406: LED5B.A R807.1
N$168
  Top 0.406: C8.2 R1.1 | R1.1 C1.2 | D-B.3 R1.1
N$169
  Top 0.406: R4.1 LED-B.A
N$170  (via drill 0.61)
  Top 0.406: R3.1 v168.91,27.94 | R29.2 C5.2 R28.1 167.85,12.38 v167,12.38 169.1,12.38 C6.2
  Bottom 0.406: v168.91,27.94 167,27.94 v167,12.38
N$171
  Top 0.406: R14.1 R9.1 IC3.5
N$172
  Top 0.406: R16.1 R11.1 IC4.5
N$173
  Top 0.406: R13.1 R6.1 IC2.5
N$174
  Top 0.406: R7.2 146.05,96.52 149.54,96.52 J2.1
N$175
  Top 0.406: R6.2 152.72,95.89 J2.2
N$176
  Top 0.406: J2.3 155.57,95.89 R8.2
N$177
  Top 0.406: J2.6 159.38,95.89 161.29,98.11 R9.2
N$178
  Top 0.406: R10.2 164.47,97.16 160.66,93.34 J2.7
N$179
  Top 0.406: R11.2 171.13,92.08 J2.8
N$180
  Top 0.406: IC2.1 147.64,106.68 | 147.64,106.68 147.64,101.92 R12.2 | R19.1 147.64,106.68
N$181
  Top 0.406: R13.2 148.91,100.23 148.91,106.36 IC2.8 R18.1
N$182
  Top 0.406: R14.2 158.75,100.23 158.75,106.36 IC3.8 R21.1
N$183
  Top 0.406: 157.48,106.68 IC3.1 | R20.1 157.48,106.68 | 157.48,106.68 157.48,101.92 R15.2
N$184
  Top 0.406: R16.2 168.59,100.23 168.59,106.36 IC4.8 R23.1
N$185
  Top 0.406: 167.32,106.68 167.32,101.92 R17.2 | 167.32,106.68 IC4.1 | R22.1 167.32,106.68
N$186
  Top 0.406: IC2.2 143.83,105.73 143.83,109.22 C10.1
N$187
  Top 0.406: IC3.2 153.67,105.73 153.67,109.22 C11.1
N$188
  Top 0.406: IC4.2 163.51,105.73 163.51,109.22 C12.1
N$189
  Top 0.406: IC5.1 144.44,90.81 142.88,90.81 142.88,88.91 IC5.3 144.44,88.9 142.88,88.9 142.88,86.72 C14.1 C13.1 149.01,88.27 156.84,88.27 | 156.84,88.27 167.74,88.27 R24.1 | J2.4 156.84,88.27
N$190
  Top 0.406: R24.2 LED-C.A
N$191  (via drill 0.61)
  Top 0.406: v166.05,107.95 R27.2
  Bottom 0.406: SJ3.1 168.91,107.95 v166.05,107.95
N$192  (via drill 0.61)
  Top 0.406: R26.2 v156.21,107.95
  Bottom 0.406: SJ2.1 159.07,107.95 v156.21,107.95
N$193  (via drill 0.61)
  Top 0.406: v146.37,107.95 R25.2
  Bottom 0.406: SJ1.1 149.22,107.95 v146.37,107.95
N$197
  Top 0.406: IC503.3 103.82,9.83 | 103.82,9.83 105.41,9.83 C506.1 | IC503.1 103.82,7.95 103.82,9.83 | C507.1 103.19,15.78 R510.2 R509.2 105.51,9.74
  Top 0.61: 105.51,9.74 C506.1
N$199
  Top 0.406: C508.1 119.79,89.95 IC502.1 123.06,87.02 | R505.2 125.09,87.02 123.06,87.02 | C509.1 123.06,87.02
N$200
  Top 0.406: F600.2 R609.1
N$201
  Top 0.406: C608.1 R608.1
N$202
  Top 0.406: F800.1 R826.2
N$203
  Top 0.406: C818.1 R831.2
N$204
  Top 0.406: R509.1 F502.2
N$205
  Top 0.406: C521.2 R510.1
N$206
  Top 0.406: R511.1 C522.2
N$207
  Top 0.406: F501.2 R508.1
N$208
  Top 0.406: C430.1 13.12,23.45 L403.2
  Top 0.813: L403.2 6.03,23.45 E-INPUT.1
N$209
  Top 0.406: R705.1 F700.2
N$210
  Top 0.406: C704.1 R704.1
N$211
  Top 0.254: R828.1 92.71,62.92 IC800.54
N$212
  Top 0.254: IC800.52 95.25,63.92 R829.1
N$213
  Top 0.254: R830.1 96.52,64.42 IC800.51
RESET  (via drill 0.3)
  Top 0.254: v119.06,59.24 114.94,59.24 114.3,58.92 IC800.14 | v119.06,53.34 119.06,51.12 122.14,51.12 R803.1 C812.1 124.78,48.9 124.78,41.27 125.37,41.27 RESET.2
  Bottom 0.254: v119.06,59.24 v119.06,53.34
  Bottom 0.305: RESET.2 RESET.1
RX
  Top 0.406: U$1.3_RXD 30.58,98.08 R701.2
S2  (via drill 0.3)
  Top 0.254: IC402.8 v47.31,26.04 | IC405.7 60.83,25.27 v61.59,26.04
  Bottom 0.254: v47.31,26.04 48.26,26.99 56.2,26.99 57.78,25.4 60.96,25.4 v61.59,26.04
S3  (via drill 0.3)
  Top 0.254: IC302.7 47.82,46.23 v48.58,46.99 | IC405.8 v60.33,26.35 | v73.03,26.99 v73.03,45.72
  Bottom 0.254: v60.33,26.35 60.96,26.99 v73.03,26.99 | v73.03,45.72 56.52,45.72 55.24,46.99 v48.58,46.99
S4  (via drill 0.3)
  Top 0.254: IC302.8 v47.31,46.99 | IC305.7 60.83,46.23 v61.59,46.99
  Bottom 0.254: v47.31,46.99 48.26,47.94 56.2,47.94 57.78,46.35 60.96,46.35 v61.59,46.99
S5  (via drill 0.3)
  Top 0.254: v73.03,47.94 v73.03,66.99 | IC202.7 47.82,67.5 v48.58,68.26 | IC305.8 v60.33,47.31
  Bottom 0.254: v48.58,68.26 55.24,68.26 56.52,66.99 v73.03,66.99 | v73.03,47.94 60.96,47.94 v60.33,47.31
S6  (via drill 0.3)
  Top 0.254: IC202.8 v47.31,68.26 | IC205.7 60.83,67.63 v61.59,68.26
  Bottom 0.254: v61.59,68.26 60.96,67.63 57.78,67.63 56.2,69.22 48.26,69.22 v47.31,68.26
S7  (via drill 0.3)
  Top 0.254: v73.03,88.58 v73.03,69.22 | IC205.8 v60.33,68.58 | IC102.7 47.82,89.09 v48.58,89.85
  Bottom 0.254: v48.58,89.85 55.24,89.85 56.52,88.58 v73.03,88.58 | v60.33,68.58 60.96,69.22 v73.03,69.22
S8  (via drill 0.3)
  Top 0.254: v47.31,89.85 IC102.8 | v61.59,89.85 60.83,89.09 IC105.7
  Bottom 0.254: v47.31,89.85 48.26,90.81 56.2,90.81 57.78,89.22 60.96,89.22 v61.59,89.85
SCK  (via drill 0.3)
  Top 0.254: v74.3,27.62 v74.3,48.58 v74.3,69.85 v74.3,91.44 | IC202.9 46.8,67.5 v46.04,68.26 | IC102.9 46.8,89.09 v46.04,89.85 | v59.05,90.17 59.82,89.66 IC105.9 | v59.05,68.58 59.82,67.82 IC205.9 | IC302.9 46.8,46.23 v46.04,46.99 | IC305.9 59.82,46.55 v59.05,47.31 | IC402.9 46.8,25.27 v46.04,26.04 | IC405.9 59.82,25.59 v59.05,26.35 | IC800.89 v105.91,41.91
  Bottom 0.254: v46.04,89.85 47.62,91.44 59.05,91.44 | 59.05,91.44 v59.05,90.17 | v46.04,68.26 47.62,69.85 59.05,69.85 | 59.05,69.85 v59.05,68.58 | v46.04,46.99 47.62,48.58 59.05,48.58 | 59.05,48.58 v59.05,47.31 | v59.05,26.35 59.05,27.62 | 59.05,27.62 47.62,27.62 v46.04,26.04 | 59.05,69.85 v74.3,69.85 | 59.05,91.44 v74.3,91.44 | 59.05,48.58 v74.3,48.58 | 59.05,27.62 v74.3,27.62 87.63,27.8 87.63,41.91 v105.91,41.91
SERIAL-RX
  Top 0.254: IC800.78 100.41,46.91 101.6,45.72 101.6,32.38 R820.1
SERIAL-TX
  Top 0.254: IC800.79 100.91,47.05 102.23,45.72 102.23,34.92 R819.1
SI  (via drill 0.3)
  Top 0.254: IC402.7 47.82,25.27 v48.58,26.04 | IC800.91 v106.91,41.91
  Bottom 0.254: v48.58,26.04 55.24,26.04 56.52,24.77 106.91,24.77 v106.91,41.91
SWCLK
  Top 0.305: IC800.76 99.41,34.92 SWD.3
SWDIO
  Top 0.305: IC800.72 95.25,53.92 93.98,52.65 93.98,37.47 SWD.2
T_OUT_1
  Top 0.254: R101.2 17.78,83.5 IC100.3
T_OUT_2
  Top 0.254: IC300.3 17.78,40.64 R301.2
T_OUT_3
  Top 0.254: IC400.3 17.78,19.69 R401.2
T_OUT_5
  Top 0.254: IC200.3 17.78,61.91 R201.2
T_OUT_7  (via drill 0.3)
  Top 0.254: 64.77,45.44 IC306.3 v65.72,47.31 | R319.2 62.87,36.51 64.77,37.78 64.77,45.44 | 64.77,45.44 63.5,45.44 C323.1 | v79.06,46.35 L304.2
  Bottom 0.254: v65.72,47.31 79.06,47.31 v79.06,46.35
TP  (via drill 0.3, 0.3 pad 0.25)
  Top 0.254: C103.1 R107.2 24.45,70.8 | 24.45,70.8 19.05,70.8 19.05,68.26 v19.37,67.94 | C203.1 R207.2 24.45,49.53 v19.37,49.53 19.05,49.21 19.05,47.62 v19.37,47.31 | C303.1 R307.2 24.45,28.26 v19.37,28.26 v19.37,25.72 | v19.37,7.3 24.45,7.3 R407.2 C403.1 | 24.45,70.8 72.07,70.8 v72.07,72.71 | IC800.29 v109.91,72.71
  Bottom 0.254: v19.37,47.31 v19.37,28.26 | v19.37,7.3 v19.37,25.72 | v19.37,67.94 v19.37,49.53 | v72.07,72.71 v109.91,72.71
TX
  Top 0.406: R700.2 27.94,95.25 26.67,96.98 U$1.2_TXD
USBD+  (via drill 0.3)
  Top 0.254: 93.34,27.94 93.34,53.15 94.61,54.42 IC800.71 | 93.34,27.94 v93.34,12.38 | R825.1 93.34,27.94
  Bottom 0.254: USB.3 7.94,10.16 7.94,4.45 93.34,4.45 v93.34,12.38
USBD-  (via drill 0.3)
  Top 0.254: v92.08,19.37 92.71,20.32 92.71,53.65 93.98,54.92 IC800.70
  Bottom 0.254: USB.2 5.59,13.02 8.89,13.02 8.89,5.08 92.08,5.08 v92.08,19.37
USBID  (via drill 0.3)
  Top 0.254: USB.4 5.59,7.3 v9.84,7.3 | v91.12,20.32 92.08,21.59 92.08,54.29 93.2,55.42 IC800.69
  Bottom 0.254: v9.84,7.3 9.84,5.71 91.12,5.71 v91.12,20.32
USBV
  Top 0.813: F500.2 11.11,5.08 11.11,9.53 8.89,9.53 8.89,20.32 POWER.1
USBV0
  Top 0.813: USB.1 6.79,17.78 POWER.2
V+  (via drill 0.3, 0.6)
  Top 0.254: R800.2 128.27,104.14 | R824.2 135.57,75.88 v133.35,75.88 | v129.54,75.88 128.24,75.88 | 123.19,20.64 131.55,20.64 131.55,24.98 R504.2 R503.2
  Top 0.406: BUZZER.- 130.81,115.57 130.81,104.14 128.27,104.14 | R505.1 128.24,79.75
  Top 0.61: R800.2 128.24,104.24 | 117.16,28.26 C511.1 | R507.1 66.99,104.14 | v99.06,26.67 114.3,26.67 | 114.3,22.86 F501.1 | 112.53,8.26 C512.1 112.55,8.26 | 112.53,15.88 F502.1
  Top 0.813: 114.3,38.1 128.24,38.1 128.24,75.88 128.24,79.75 v128.24,101.6 128.24,104.24 | 114.3,38.1 114.3,28.36 | SERIAL.1 114.3,40.01 114.3,38.1 | v118.11,101.6 v108.9,101.6 R506.1 | C501.1 117.16,28.26 123.19,28.26 C520.+ 123.19,20.64 123.19,17.78 119.38,17.78 | C511.1 114.3,28.36 | 66.99,104.14 66.99,101.6 v69.16,101.6 | 114.3,28.36 114.3,26.67 114.3,22.86 114.3,17.78 | F502.1 114.3,15.88 114.3,17.78 | 112.53,8.26 C500.1 | C500.1 112.53,15.88 | C500.1 C519.+ | 112.55,8.26 F500.1 119.38,5.08 C519.+ | 119.38,17.78 114.3,17.78 | 119.38,17.78 C519.+
  Bottom 0.254: v133.35,75.88 v129.54,75.88 | 96.52,26.67 91.44,26.67 J3.1
  Bottom 0.61: v99.06,26.67 96.52,26.67 SWD.5
  Bottom 0.813: v118.11,101.6 v128.24,101.6 | v69.16,101.6 v108.9,101.6
V+B
  Top 0.406: D-B.2 R4.2 C4.2 161.93,23.62 | IC1.5 159.35,23.62 161.93,23.62 | R28.2 C3.2 161.93,17.14 161.93,19.05 | 161.93,23.62 161.93,19.05 | L1.1 161.93,19.05
VDD  (via drill 0.3, 0.5, 0.6 pad 0.25)
  Top 0.254: IC405.10 59.33,24.21 C422.2 v57.47,22.23 | IC406.5 C425.2 v67.94,17.46 | IC105.10 59.33,88.03 C122.2 v57.47,86.04 | IC106.5 C125.2 v67.94,81.28 | IC206.5 C225.2 v67.94,59.69 | IC205.10 59.33,66.44 C222.2 v57.47,64.45 | IC101.5 41.59,86.99 C112.2 42.86,88.9 | IC305.10 59.33,45.16 C322.2 v57.47,43.18 | IC306.5 C325.2 v67.94,38.42 | v20.64,67.94 20.64,65.72 | 20.64,65.72 20.64,63.81 IC200.5 | 42.86,88.9 v42.86,90.81 | 42.86,46.04 v42.86,47.94 | 42.86,25.08 C415.2 IC401.5 | 42.86,25.08 v42.86,26.99 | v20.64,89.53 20.64,87 | 20.64,87 20.64,85.41 IC100.5 | v20.64,46.67 20.64,44.45 | 20.64,44.45 20.64,42.54 IC300.5 | v20.64,25.72 20.64,23.5 | 20.64,23.5 20.64,21.59 IC400.5 | 42.86,25.08 C412.2 46.32,24.23 IC402.10 | C402.2 20.64,23.5 | C302.2 20.64,44.45 | C202.2 20.64,65.72 | C102.2 20.64,87 | 42.86,46.04 C312.2 46.32,45.19 IC302.10 | 42.86,46.04 C315.2 IC301.5 | IC202.10 46.32,66.46 C212.2 42.86,67.31 | IC102.10 46.32,88.05 C115.2 42.86,88.9 | IC201.5 C215.2 42.86,67.31 | v42.86,69.22 42.86,67.31
  Top 0.406: v77.15,83.19 v77.15,61.59 v77.15,40.32 v77.15,19.37 77.15,7.94 C504.1 IC501.5 | v85.44,83.19 IC500.5
  Bottom 0.254: v20.64,89.53 20.64,90.81 v42.86,90.81 | v20.64,67.94 20.64,69.22 v42.86,69.22 | v20.64,46.67 20.64,47.94 v42.86,47.94
  Bottom 0.406: v42.86,69.22 47.31,64.77 49.21,64.77 49.85,65.41 56.52,65.41 v57.47,64.45 60.01,61.59 67.94,61.59 | v42.86,90.81 47.31,86.36 49.21,86.36 49.85,87 56.52,87 v57.47,86.04 60.01,83.19 67.94,83.19 | 67.94,61.59 v67.94,59.69 | 67.94,61.59 v77.15,61.59 | v42.86,47.94 47.31,43.5 49.21,43.5 49.85,44.13 56.52,44.13 v57.47,43.18 60.01,40.32 67.94,40.32 | 67.94,83.19 v67.94,81.28 | v67.94,38.42 67.94,40.32 | 67.94,40.32 v77.15,40.32 | 67.94,19.37 60.01,19.37 v57.47,22.23 56.52,23.18 49.53,23.18 48.9,22.54 47.31,22.54 v42.86,26.99 20.64,26.99 v20.64,25.72 | 67.94,19.37 v67.94,17.46 | 67.94,83.19 v77.15,83.19 v85.44,83.19 | 67.94,19.37 v77.15,19.37
VREF  (via drill 0.5)
  Top 0.254: C806.1 124.88,64.77 119.06,64.77 119.06,62.42 IC800.21
  Top 0.406: C806.1 C808.1 124.88,72.39 | 124.88,72.39 v124.88,75.03 | 124.88,72.39 R804.2 | R500.1 86.68,75.03 v86.68,74.93
  Bottom 0.406: v86.68,74.93 v124.88,75.03

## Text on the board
tPlace: * | H-Amp 1 | * | * | * | * | * | * | * | * | * | *
tNames: 25 MHz | Blitzortung.org - PCB 16.2 - 2021-03-31 | 25 MHz | H-Amp 2 | 8 MHz | GND | H-Amp 3 | Blitzortung.org - PCB 17.3 - 2022-01-10 | E-Amp | Blitzortung.org - System Blue / PCB 20.8 - 2022.05.02 | Blitzortung.org - PCB 19.7 - 2022-01-10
